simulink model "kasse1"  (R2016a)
settings: Solver=FixedStepDiscrete  StartTime=0.0  StopTime=100  FixedStep=0.001  MaxStep=0.01  RelTol=1e-3
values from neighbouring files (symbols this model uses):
  lambda = block.DialogPrm(1).Data    [sfun_poisson.m]
undefined symbols (not defined in the file or in its folder): tAb, z0
libraries: simulink x2

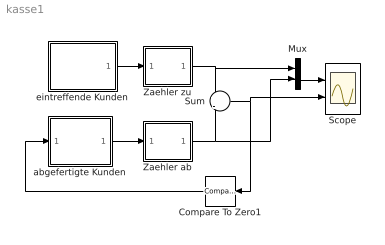
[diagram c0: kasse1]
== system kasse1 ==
  Compare To Zero1 : simulink/Logic and Bit Operations/Compare To Zero  relop=<=  OutDataTypeStr=uint8
  Mux : Mux  Inputs=2
  Scope : Scope  NumInputPorts=2
  Sum : Sum  Inputs=+|-
  Zaehler ab : Subsystem
  Zaehler zu : Subsystem
  abgefertigte Kunden : Subsystem
  eintreffende Kunden : Subsystem
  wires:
  Zaehler zu/1(Out) -> Sum/1, Mux/1
  eintreffende Kunden/1(Out) -> Zaehler zu/1(In)
  abgefertigte Kunden/1(Out) -> Zaehler ab/1(In)
  Zaehler ab/1(Out) -> Sum/2, Mux/2
  Sum/1 -> Compare To Zero1/1, Scope/2
  Compare To Zero1/1 -> abgefertigte Kunden/1(In1)
  Mux/1 -> Scope/1

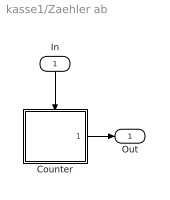
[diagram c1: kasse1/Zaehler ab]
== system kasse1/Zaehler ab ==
  In : Inport
  Counter : Subsystem
  Out : Outport
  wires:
  Counter/1(Out) -> Out/1
  In/1 -> Counter/Trigger

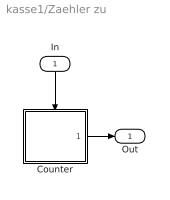
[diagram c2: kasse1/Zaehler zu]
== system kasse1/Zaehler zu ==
  In : Inport
  Counter : Subsystem
  Out : Outport
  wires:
  Counter/1(Out) -> Out/1
  In/1 -> Counter/Trigger

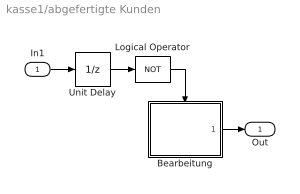
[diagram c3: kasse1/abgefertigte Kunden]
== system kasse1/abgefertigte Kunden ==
  In1 : Inport
  Bearbeitung : Subsystem
  Logical Operator : Logic  Operator=NOT  AllPortsSameDT=off  OutDataTypeStr=boolean
  Unit Delay : UnitDelay  SampleTime=-1
  Out : Outport
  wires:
  Bearbeitung/1(Out) -> Out/1
  In1/1 -> Unit Delay/1
  Unit Delay/1 -> Logical Operator/1
  Logical Operator/1 -> Bearbeitung/Enable

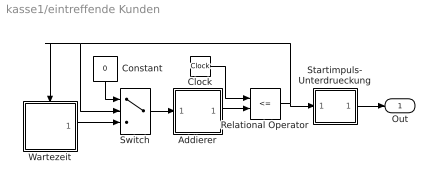
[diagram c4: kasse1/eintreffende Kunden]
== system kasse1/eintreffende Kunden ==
  Addierer : Subsystem
  Clock : Clock
  Constant : Constant  Value=0
  Relational Operator : RelationalOperator  Operator=<=  OutDataTypeStr=boolean
  Startimpuls- Unterdrueckung : Subsystem
  Switch : Switch  Threshold=1
  Wartezeit : Subsystem
  Out : Outport
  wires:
  Clock/1 -> Relational Operator/1
  Relational Operator/1 -> Switch/2, Wartezeit/Trigger, Startimpuls- Unterdrueckung/1(In)
  Addierer/1(Summe) -> Relational Operator/2
  Switch/1 -> Addierer/1(In)
  Wartezeit/1(dt) -> Switch/3
  Constant/1 -> Switch/1
  Startimpuls- Unterdrueckung/1(Out) -> Out/1

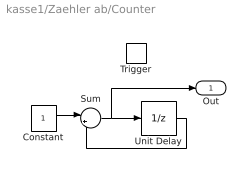
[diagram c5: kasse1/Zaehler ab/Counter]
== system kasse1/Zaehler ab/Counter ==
  Trigger : TriggerPort  TriggerType=falling  VariantControl=Variant
  Constant : Constant
  Sum : Sum  Inputs=|++
  Unit Delay : UnitDelay  InitialCondition=z0  SampleTime=-1
  Out : Outport  InitialOutput=z0
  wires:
  Constant/1 -> Sum/1
  Sum/1 -> Unit Delay/1, Out/1
  Unit Delay/1 -> Sum/2

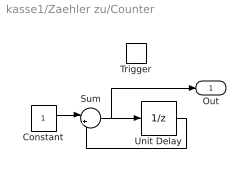
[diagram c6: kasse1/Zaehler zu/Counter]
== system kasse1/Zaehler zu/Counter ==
  Trigger : TriggerPort  TriggerType=falling  VariantControl=Variant
  Constant : Constant
  Sum : Sum  Inputs=|++
  Unit Delay : UnitDelay  InitialCondition=z0  SampleTime=-1
  Out : Outport  InitialOutput=z0
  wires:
  Constant/1 -> Sum/1
  Sum/1 -> Unit Delay/1, Out/1
  Unit Delay/1 -> Sum/2

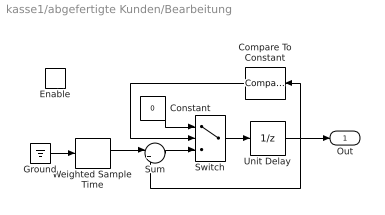
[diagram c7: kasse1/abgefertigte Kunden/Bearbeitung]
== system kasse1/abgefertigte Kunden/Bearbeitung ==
  Enable : EnablePort  StatesWhenEnabling=reset
  Compare To Constant : simulink/Logic and Bit Operations/Compare To Constant  SystemSampleTime=-1  relop=>=  const=tAb  LogicOutDataTypeMode=uint8
  Constant : Constant  Value=0
  Ground : Ground
  Sum : Sum  Inputs=|++
  Switch : Switch  Threshold=1
  Unit Delay : UnitDelay  SampleTime=-1
  Weighted Sample Time : SampleTimeMath  TsampMathOp=Ts Only  weightValue=1
  Out : Outport  OutputWhenDisabled=reset  InitialOutput=0
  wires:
  Compare To Constant/1 -> Switch/2
  Constant/1 -> Switch/1
  Switch/1 -> Unit Delay/1
  Sum/1 -> Switch/3
  Weighted Sample Time/1 -> Sum/1
  Ground/1 -> Weighted Sample Time/1
  Unit Delay/1 -> Compare To Constant/1, Sum/2, Out/1

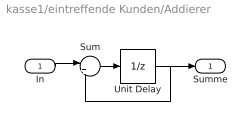
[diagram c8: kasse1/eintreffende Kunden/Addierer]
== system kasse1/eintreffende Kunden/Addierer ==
  In : Inport
  Sum : Sum  Inputs=|++
  Unit Delay : UnitDelay  SampleTime=-1
  Summe : Outport
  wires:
  Sum/1 -> Unit Delay/1
  Unit Delay/1 -> Summe/1, Sum/2
  In/1 -> Sum/1

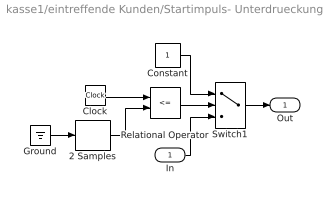
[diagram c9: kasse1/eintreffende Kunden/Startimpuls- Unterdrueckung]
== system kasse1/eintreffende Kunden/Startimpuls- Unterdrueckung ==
  In : Inport
  2 Samples : SampleTimeMath  TsampMathOp=Ts Only  weightValue=2
  Clock : Clock
  Constant : Constant
  Ground : Ground
  Relational Operator : RelationalOperator  Operator=<=  OutDataTypeStr=boolean
  Switch1 : Switch  Threshold=1
  Out : Outport
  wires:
  In/1 -> Switch1/3
  Constant/1 -> Switch1/1
  Relational Operator/1 -> Switch1/2
  Switch1/1 -> Out/1
  Clock/1 -> Relational Operator/1
  2 Samples/1 -> Relational Operator/2
  Ground/1 -> 2 Samples/1

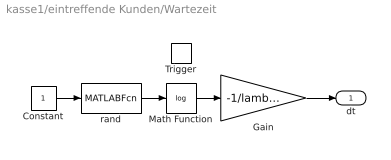
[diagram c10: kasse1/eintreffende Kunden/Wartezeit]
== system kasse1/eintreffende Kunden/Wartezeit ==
  Trigger : TriggerPort  TriggerType=falling  VariantControl=Variant
  Constant : Constant
  Gain : Gain  Gain=-1/lambda
  Math Function : Math  Operator=log
  rand : MATLABFcn  MATLABFcn=rand
  dt : Outport
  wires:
  Constant/1 -> rand/1
  Gain/1 -> dt/1
  Math Function/1 -> Gain/1
  rand/1 -> Math Function/1
